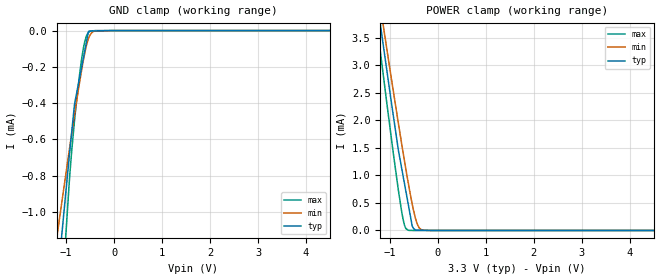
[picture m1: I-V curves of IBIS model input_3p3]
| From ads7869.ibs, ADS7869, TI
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|   input_3p3 Model
[Model]   input_3p3
Model_type   Input
Vinl = 0.8
Vinh = 2.0
|   typ   min   max
|   (nom PVT)   (fast PVT)   (slow PVT)
|C_comp from frequency sweep method (F=16MHz)
|Average
|C_comp   2.315e-12   2.232e-12   2.398e-12
|C_comp from LC tank measurement(L=1nH)
|Average
|Resonant Frequency(Hz)   3.610e+09   3.650e+09   3.560e+09
C_comp   1.946e-12   1.903e-12   2.001e-12
| Where nom  PVT is Nominal Process, 3.3V, 36C
|   Fast PVT is Strong Process,  3.6V, -40C
|   Slow PVT is Weak Process,   3V, 96C
[Voltage Range]   3.3   3   3.6
|Ambient Temperature   25   85   -40
|Junction Temperature
[Temperature Range]   36   96   -40
[Power Clamp Reference]   3.3   3   3.6
[GND Clamp Reference]   0   0   0
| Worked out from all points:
|   GND clamp passes 1 mA (typ) near -1.04 V on its own axis
|   POWER clamp passes 1 mA (typ) near -0.73 V on its own axis
[GND Clamp]
|   Voltage   I(typ)   I(min)   I(max)
-3.3V     -7.702mA   -5.247mA   -13.6mA
-1.165V   -1.344mA   -1.088mA   -1.885mA
-1.089V   -1.123mA   -945.9uA   -1.517mA
-1.018V   -924.1uA   -813.7uA   -1.174mA
-877.2mV  -543.5uA   -556.9uA   -644.4uA
-825mV    -406.8uA   -463.8uA   -497.3uA
-726mV    -269.8uA   -295.4uA   -255.9uA
-639.6mV  -150.3uA   -163.3uA   -96.29uA
-534.6mV  -4.947uA   -44.53uA   -10.53uA
-414mV    -2.169uA   -2.876uA   -648.6nA
-28.87fV  0A         0A         0A
6.6V      0A         0A         0A
[POWER Clamp]
|   Voltage   I(typ)   I(min)   I(max)
-3.3V     17.16mA    16.43mA    18.25mA
-1.259V   4.122mA    4.413mA    3.661mA
-1.167V   3.545mA    3.881mA    3.026mA
-1.135V   3.346mA    3.7mA      2.805mA
-825mV    1.469mA    1.956mA    743.9uA
-754.8mV  1.133mA    1.577mA    345.2uA
-679.2mV  771.9uA    1.18mA     57.24uA
-610.8mV  444.9uA    835uA      2.263uA
-531.3mV  73.95uA    465.9uA    478.2nA
-429mV    6.938uA    115.8uA    0A
-339mV    5.065uA    11.41uA    0A
6.6V      0A         0A         0A
